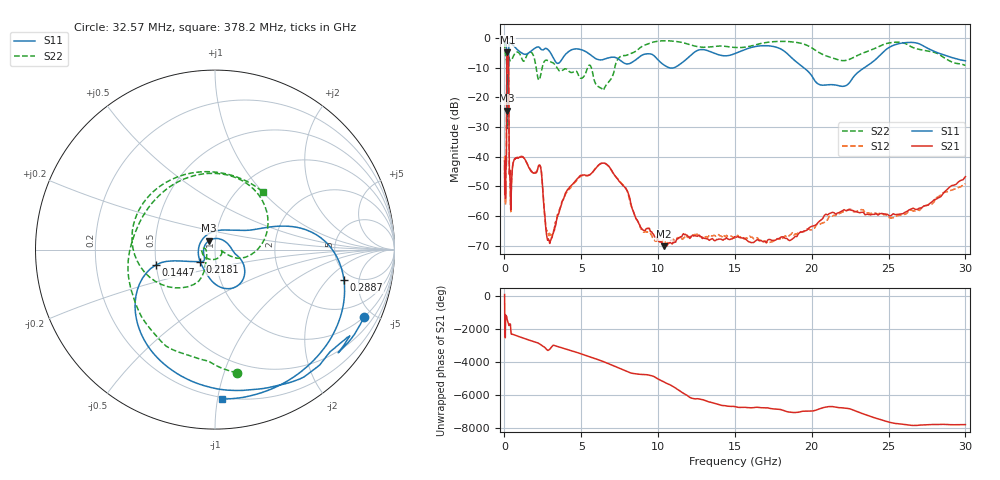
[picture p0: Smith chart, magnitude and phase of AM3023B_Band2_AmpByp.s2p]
# Hz S DB R 50.0
!freq dBS11 angS11 dBS21 angS21 dBS12 angS12 dBS22 angS22
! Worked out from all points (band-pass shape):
!   1601 points, 10 MHz to 30 GHz, reference 50 ohm
!   highest |S21| = -4.85 dB at 188.7 MHz (marker M1); lowest = -70.1 dB at 10.38 GHz (marker M2)
!   |S21| within 3 dB of the highest: 152.6 MHz to 258.7 MHz (106.1 MHz wide, 51.6 % of centre)
!   lowest |S11| = -24.5 dB at 171.5 MHz (marker M3), VSWR 1.13, Z = 46.6 + j4.7 ohm
!   |S11| at or under -10 dB: 145.2 MHz to 259 MHz (113.8 MHz wide, 56.3 % of centre); 10.72 GHz to 11.03 GHz (314.2 MHz wide, 2.89 % of centre); 19.48 GHz to 23.42 GHz (3.935 GHz wide, 18.3 % of centre)
!   |S22| runs from -30.4 to -0.9 dB; largest |S21 - S12| = 0.014
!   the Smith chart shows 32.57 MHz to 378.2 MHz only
!   S11 on the Smith chart (normalised r, x): 32.57 MHz: 1.02, -4.45; 144.7 MHz: 0.50, -0.10; 218.1 MHz: 0.84, -0.12; 288.7 MHz: 4.21, -3.14; 378.2 MHz: 0.19, -1.03
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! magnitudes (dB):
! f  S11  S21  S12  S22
! 10 MHz  -0.8  -41.5  -40.0  -1.6
! 32.57 MHz  -0.8  -49.2  -48.7  -3.1
! 38.04 MHz  -0.8  -49.0  -49.4  -3.7
! 122.1 MHz  -2.6  -42.6  -43.2  -7.3
! 144.7 MHz  -9.4  -13.7  -13.7  -9.2
! 171.5 MHz  -24.5  -5.2  -5.1  -29.3
! 188.7 MHz  -14.4  -4.9  -4.8  -24.6
! 218.1 MHz  -19.4  -5.1  -5.0  -22.6
! 258.6 MHz  -10.1  -7.8  -7.7  -18.0
! 288.7 MHz  -2.6  -25.3  -25.2  -6.4
! 315.9 MHz  -1.7  -44.4  -44.5  -6.9
! 378.2 MHz  -1.6  -49.5  -50.5  -7.6
! 547.7 MHz  -2.4  -42.5  -42.3  -6.5
! 2.084 GHz  -3.1  -45.3  -45.1  -10.8
! 2.361 GHz  -3.7  -43.8  -43.5  -12.3
! 2.899 GHz  -4.3  -68.0  -66.6  -7.8
! 6.234 GHz  -7.4  -42.4  -42.4  -16.7
! 7.926 GHz  -8.7  -50.9  -50.8  -5.8
! 10.38 GHz  -9.1  -70.1  -68.2  -0.9
! 18.28 GHz  -4.7  -67.5  -66.6  -1.1
! 21.35 GHz  -15.7  -58.7  -60.0  -6.7
! 30 GHz  -7.7  -46.7  -49.1  -9.2
